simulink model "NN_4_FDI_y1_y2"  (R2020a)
settings: Solver=VariableStepAuto  StartTime=0.0  StopTime=30  RelTol=1e-3
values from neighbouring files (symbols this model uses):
  C = 6.3000e-04    (= 0.00063)    [maglev_init.m]
  g = 9.80    (= 9.8)    [maglev_init.m]
  K = 1.0e+03 * [-2.4567   -0.1235    0.0237]    [maglev_init.m]
  L1 = 0.6000    (= 0.6)    [maglev_init.m]
  m = 0.0300    (= 0.03)    [maglev_init.m]
  mpert = 0    [maglev_init.m]
  R = 45    [maglev_init.m]
  Ts = 0.005    [maglev_init.m]    (also in train_net.m)
  x1_0 = 0.1    [maglev_init.m]
  x1_d = 0.05    [maglev_init.m]
  x2_0 = 0    [maglev_init.m]
  x2_d = 0    [maglev_init.m]
  x3_0 = 0.2    [maglev_init.m]
libraries: neural x36

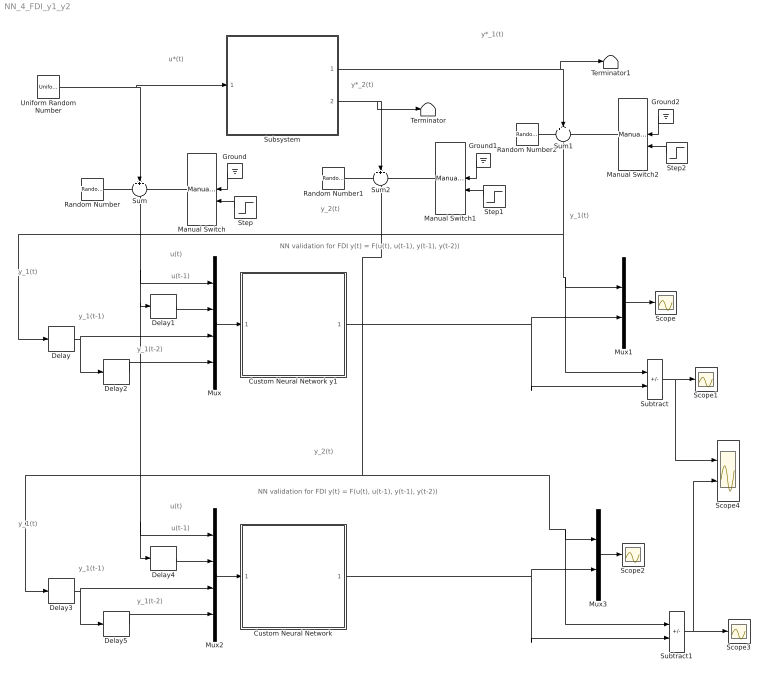
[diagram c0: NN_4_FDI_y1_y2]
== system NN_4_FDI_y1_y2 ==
  note: y_1(t)
  note: y_1(t-1)
  note: NN validation for FDI y(t) = F(u(t), u(t-1), y(t-1), y(t-2))
  note: y_2(t)
  note: y*_1(t)
  note: u(t)
  note: u*(t)
  note: y*_2(t)
  note: y_1(t)
  note: u(t-1)
  note: y_1(t-2)
  note: y_1(t)
  note: y_1(t-1)
  note: u(t-1)
  note: NN validation for FDI y(t) = F(u(t), u(t-1), y(t-1), y(t-2))
  note: u(t)
  note: y_1(t-2)
  note: y_2(t)
  Custom Neural Network : Subsystem
      mask help: Custom Neural Network
  Custom Neural Network y1 : Subsystem
      mask help: Custom Neural Network
  Delay{,1..5} (6 alike) : Delay  DelayLength=1  SampleTime=Ts
  Ground : Ground
  Ground1 : Ground
  Ground2 : Ground
  Manual Switch : ManualSwitch
  Manual Switch1 : ManualSwitch
  Manual Switch2 : ManualSwitch
  Mux : Mux
  Mux1 : Mux  Inputs=2
  Mux2 : Mux
  Mux3 : Mux  Inputs=2
  Random Number : RandomNumber  Variance=1e-9  Seed=1  SampleTime=Ts
  Random Number1 : RandomNumber  Variance=1e-6  Seed=3  SampleTime=Ts
  Random Number2 : RandomNumber  Variance=1e-9  Seed=2  SampleTime=Ts
  Scope{,1..3} (4 alike) : Scope
  Scope4 : Scope  NumInputPorts=2
  Step : Step  Time=15  SampleTime=0
  Step1 : Step  Time=15  After=5  SampleTime=0
  Step2 : Step  Time=15  SampleTime=0
  Subsystem : Subsystem
  Subtract : Sum  Inputs=+-
  Subtract1 : Sum  Inputs=+-
  Sum : Sum  Inputs=+++
  Sum1 : Sum  Inputs=+++
  Sum2 : Sum  Inputs=+++
  Terminator : Terminator
  Terminator1 : Terminator
  Uniform Random Number : UniformRandomNumber  Minimum=x1_d*0.9  Maximum=x1_d*1.1  Seed=1  SampleTime=0.5
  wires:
  Uniform Random Number/1 -> Subsystem/1(In1), Sum/2
  Subsystem/1(Out1) -> Terminator1/1, Sum1/2
  Subsystem/2(Out2) -> Terminator/1, Sum2/2
  Random Number/1 -> Sum/1
  Manual Switch/1 -> Sum/3
  Manual Switch2/1 -> Sum1/3
  Manual Switch1/1 -> Sum2/3
  Random Number1/1 -> Sum2/1
  Ground/1 -> Manual Switch/1
  Step/1 -> Manual Switch/2
  Ground1/1 -> Manual Switch1/1
  Step1/1 -> Manual Switch1/2
  Random Number2/1 -> Sum1/1
  Ground2/1 -> Manual Switch2/1
  Step2/1 -> Manual Switch2/2
  Sum1/1 -> Subtract/1, Mux1/1, Delay/1
  Delay1/1 -> Mux/2
  Delay/1 -> Delay2/1, Mux/3
  Delay2/1 -> Mux/4
  Mux/1 -> Custom Neural Network y1/1(Input)
  Custom Neural Network y1/1(Output) -> Subtract/2, Mux1/2
  Mux1/1 -> Scope/1
  Subtract/1 -> Scope4/1, Scope1/1
  Delay5/1 -> Mux2/4
  Mux3/1 -> Scope2/1
  Custom Neural Network/1(Output) -> Subtract1/2, Mux3/2
  Mux2/1 -> Custom Neural Network/1(Input)
  Delay3/1 -> Delay5/1, Mux2/3
  Sum/1 -> Delay4/1, Mux2/1, Delay1/1, Mux/1
  Delay4/1 -> Mux2/2
  Subtract1/1 -> Scope4/2, Scope3/1
  Sum2/1 -> Subtract1/1, Mux3/1, Delay3/1

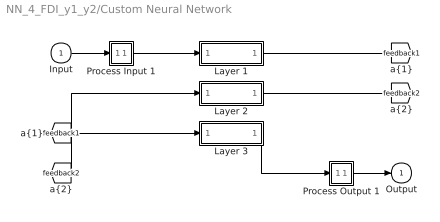
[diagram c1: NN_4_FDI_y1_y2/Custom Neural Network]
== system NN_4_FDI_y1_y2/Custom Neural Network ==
  Input : Inport  PortDimensions=4  SampleTime=0.005
  Layer 1 : Subsystem
  Layer 2 : Subsystem
  Layer 3 : Subsystem
  Process Input 1 : Subsystem
  Process Output 1 : Subsystem
  Output : Outport  InitialOutput=0
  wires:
  Input/1 -> Process Input 1/1(x)
  Process Output 1/1(y) -> Output/1
  Process Input 1/1(p) -> Layer 1/1("p{1}")
  Layer 1/1("a{1}") -> [feedback1]
  [feedback1] -> Layer 2/1("a{1} ")
  Layer 2/1("a{2}") -> [feedback2]
  [feedback2] -> Layer 3/1("a{2} ")
  Layer 3/1("a{3}") -> Process Output 1/1(a)

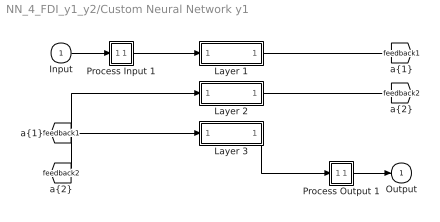
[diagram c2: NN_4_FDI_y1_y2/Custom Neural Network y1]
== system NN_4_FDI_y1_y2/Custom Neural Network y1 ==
  Input : Inport  PortDimensions=4  SampleTime=0.005
  Layer 1 : Subsystem
  Layer 2 : Subsystem
  Layer 3 : Subsystem
  Process Input 1 : Subsystem
  Process Output 1 : Subsystem
  Output : Outport  InitialOutput=0
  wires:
  Input/1 -> Process Input 1/1(x)
  Process Output 1/1(y) -> Output/1
  Process Input 1/1(p) -> Layer 1/1("p{1}")
  Layer 1/1("a{1}") -> [feedback1]
  [feedback1] -> Layer 2/1("a{1} ")
  Layer 2/1("a{2}") -> [feedback2]
  [feedback2] -> Layer 3/1("a{2} ")
  Layer 3/1("a{3}") -> Process Output 1/1(a)

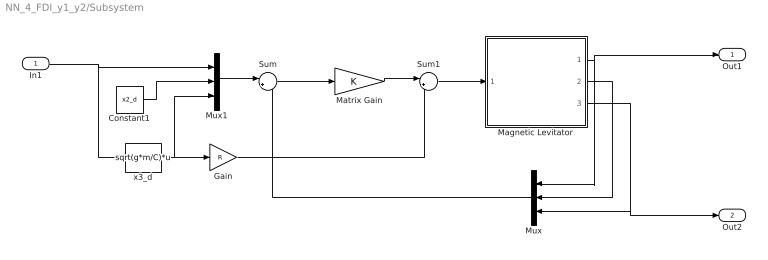
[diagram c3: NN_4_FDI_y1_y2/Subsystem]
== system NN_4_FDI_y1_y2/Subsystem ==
  In1 : Inport
  Constant1 : Constant  Value=x2_d
  Gain : Gain  Gain=R
  Magnetic Levitator : Subsystem  mask{m=m+mpert, R=R, L1=L1, C=C, g=g}
      mask prompts: m "ball's mass (m)"; R "Electromagnet's resistance (R)"; L1 "Electromagnet's inductance (L1)"; C "Magnetic force constant (C)"; g "Gravitational acceleration (g)"
  Matrix Gain : Gain  Gain=K  Multiplication=Matrix(K*u)  SaturateOnIntegerOverflow=on
  Mux : Mux  Inputs=3
  Mux1 : Mux  Inputs=3
  Sum : Sum  Inputs=|+-  InputSameDT=on  SaturateOnIntegerOverflow=on
  Sum1 : Sum  Inputs=|++  InputSameDT=on  SaturateOnIntegerOverflow=on
  x3_d : Fcn  Expr=sqrt(g*m/C)*u
  Out1 : Outport
  Out2 : Outport  Port=2
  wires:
  In1/1 -> x3_d/1, Mux1/1
  Magnetic Levitator/2(x2) -> Mux/2
  x3_d/1 -> Mux1/3, Gain/1
  Mux1/1 -> Sum/1
  Gain/1 -> Sum1/2
  Mux/1 -> Sum/2
  Constant1/1 -> Mux1/2
  Sum/1 -> Matrix Gain/1
  Sum1/1 -> Magnetic Levitator/1(u)
  Magnetic Levitator/1(x1) -> Out1/1, Mux/1
  Magnetic Levitator/3(x3) -> Out2/1, Mux/3
  Matrix Gain/1 -> Sum1/1

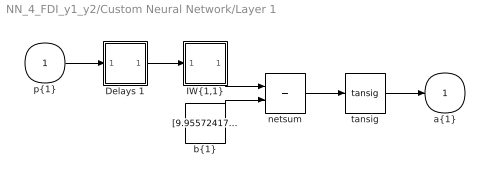
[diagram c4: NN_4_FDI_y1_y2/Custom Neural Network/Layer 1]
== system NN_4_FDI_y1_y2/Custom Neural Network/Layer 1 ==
  "p{1}" : Inport  PortDimensions=4  SampleTime=0.005
  Delays 1 : Subsystem
  "IW{1,1}" : Subsystem
  "b{1}" : Constant  Value=[9.9557241726304166462568900897167623043060302734375;10.8017518649547294984358813962899148464202880859375;3.779362190875286131586108240298926830291748046875;13.70534100885252115631374181248247623443603515625]
  netsum : Sum  Inputs=2  InputSameDT=on  SaturateOnIntegerOverflow=on
  tansig : neural/Transfer Functions/tansig
  "a{1}" : Outport  InitialOutput=[0;0;0;0]
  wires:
  "p{1}"/1 -> Delays 1/1("p{1}")
  Delays 1/1("pd{1,1}") -> "IW{1,1}"/1("pd{1,1}")
  "IW{1,1}"/1("iz{1,1}") -> netsum/1
  "b{1}"/1 -> netsum/2
  netsum/1 -> tansig/1
  tansig/1 -> "a{1}"/1

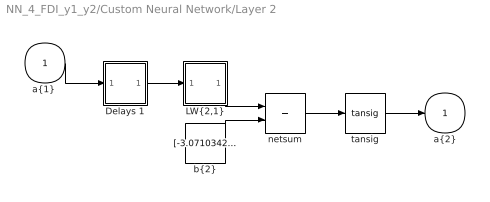
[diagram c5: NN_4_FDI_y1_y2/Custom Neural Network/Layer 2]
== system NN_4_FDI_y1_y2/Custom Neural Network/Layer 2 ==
  "a{1} " : Inport  PortDimensions=4  SampleTime=0.005
  Delays 1 : Subsystem
  "LW{2,1}" : Subsystem
  "b{2}" : Constant  Value=[-3.071034257137068568255244827014394104480743408203125;1.6519477133200834995108152725151740014553070068359375;2.0170506290868939203164700302295386791229248046875;-0.93388372923963192118179676981526426970958709716796875;0.3845725321207089653086086400435306131839752197265625;-0.39336279890520386981478395682643167674541473388671875;0.930508654862947093278080501477234065532684326171875;1.911370482300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
  netsum : Sum  Inputs=2  InputSameDT=on  SaturateOnIntegerOverflow=on
  tansig : neural/Transfer Functions/tansig
  "a{2}" : Outport  InitialOutput=[0;0;0;0;0;0;0;0;0;0]
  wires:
  "a{1} "/1 -> Delays 1/1("p{2}")
  Delays 1/1("pd{2,1}") -> "LW{2,1}"/1("ad{2,1}")
  "LW{2,1}"/1("lz{2,1}") -> netsum/1
  "b{2}"/1 -> netsum/2
  netsum/1 -> tansig/1
  tansig/1 -> "a{2}"/1

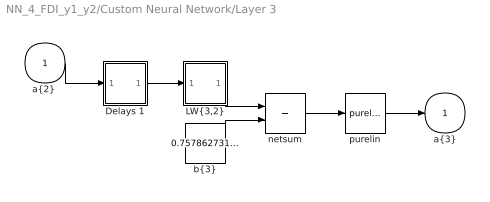
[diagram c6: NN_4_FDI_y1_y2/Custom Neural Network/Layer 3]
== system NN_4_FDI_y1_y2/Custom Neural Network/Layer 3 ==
  "a{2} " : Inport  PortDimensions=10  SampleTime=0.005
  Delays 1 : Subsystem
  "LW{3,2}" : Subsystem
  "b{3}" : Constant  Value=0.7578627315964741040232865998405031859874725341796875
  netsum : Sum  Inputs=2  InputSameDT=on  SaturateOnIntegerOverflow=on
  purelin : neural/Transfer Functions/purelin
  "a{3}" : Outport  InitialOutput=0
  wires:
  "a{2} "/1 -> Delays 1/1("p{3}")
  Delays 1/1("pd{3,2}") -> "LW{3,2}"/1("ad{3,2}")
  "LW{3,2}"/1("lz{3,2}") -> netsum/1
  "b{3}"/1 -> netsum/2
  netsum/1 -> purelin/1
  purelin/1 -> "a{3}"/1

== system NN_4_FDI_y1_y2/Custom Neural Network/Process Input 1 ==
  x : Inport  PortDimensions=4  SampleTime=0.005
  p : Outport  PortDimensions=4  SampleTime=0.005
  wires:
  x/1 -> p/1

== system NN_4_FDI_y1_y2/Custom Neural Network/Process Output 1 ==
  a : Inport  PortDimensions=1  SampleTime=0.005
  y : Outport  PortDimensions=1  SampleTime=0.005
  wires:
  a/1 -> y/1

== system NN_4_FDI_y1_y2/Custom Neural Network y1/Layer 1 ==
  "p{1}" : Inport  PortDimensions=4  SampleTime=0.005
  Delays 1 : Subsystem
  "IW{1,1}" : Subsystem
  "b{1}" : Constant  Value=[11.744601348517022643136442638933658599853515625;10.199640082309191058129727025516331195831298828125;-17.03232759988026856490250793285667896270751953125;13.5748992182948189366697988589294254779815673828125]
  netsum : Sum  Inputs=2  InputSameDT=on  SaturateOnIntegerOverflow=on
  tansig : neural/Transfer Functions/tansig
  "a{1}" : Outport  InitialOutput=[0;0;0;0]
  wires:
  "p{1}"/1 -> Delays 1/1("p{1}")
  Delays 1/1("pd{1,1}") -> "IW{1,1}"/1("pd{1,1}")
  "IW{1,1}"/1("iz{1,1}") -> netsum/1
  "b{1}"/1 -> netsum/2
  netsum/1 -> tansig/1
  tansig/1 -> "a{1}"/1

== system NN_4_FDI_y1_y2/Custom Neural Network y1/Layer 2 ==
  "a{1} " : Inport  PortDimensions=4  SampleTime=0.005
  Delays 1 : Subsystem
  "LW{2,1}" : Subsystem
  "b{2}" : Constant  Value=[2.514902413299356709330822923220694065093994140625;-1.905736181055616373924976869602687656879425048828125;-1.3244117236339700838243516045622527599334716796875;1.4169478908980768228076385639724321663379669189453125;-0.54494294986358460253228486180887557566165924072265625;0.1603376935224779253896798536516143940389156341552734375;-0.8398255160686165510242062737233936786651611328125;-1.30541599158430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
  netsum : Sum  Inputs=2  InputSameDT=on  SaturateOnIntegerOverflow=on
  tansig : neural/Transfer Functions/tansig
  "a{2}" : Outport  InitialOutput=[0;0;0;0;0;0;0;0;0;0]
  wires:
  "a{1} "/1 -> Delays 1/1("p{2}")
  Delays 1/1("pd{2,1}") -> "LW{2,1}"/1("ad{2,1}")
  "LW{2,1}"/1("lz{2,1}") -> netsum/1
  "b{2}"/1 -> netsum/2
  netsum/1 -> tansig/1
  tansig/1 -> "a{2}"/1

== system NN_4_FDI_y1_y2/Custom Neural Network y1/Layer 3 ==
  "a{2} " : Inport  PortDimensions=10  SampleTime=0.005
  Delays 1 : Subsystem
  "LW{3,2}" : Subsystem
  "b{3}" : Constant  Value=-0.57244236899128775331035967610660009086132049560546875
  netsum : Sum  Inputs=2  InputSameDT=on  SaturateOnIntegerOverflow=on
  purelin : neural/Transfer Functions/purelin
  "a{3}" : Outport  InitialOutput=0
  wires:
  "a{2} "/1 -> Delays 1/1("p{3}")
  Delays 1/1("pd{3,2}") -> "LW{3,2}"/1("ad{3,2}")
  "LW{3,2}"/1("lz{3,2}") -> netsum/1
  "b{3}"/1 -> netsum/2
  netsum/1 -> purelin/1
  purelin/1 -> "a{3}"/1

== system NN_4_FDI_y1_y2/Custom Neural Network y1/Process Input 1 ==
  x : Inport  PortDimensions=4  SampleTime=0.005
  p : Outport  PortDimensions=4  SampleTime=0.005
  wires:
  x/1 -> p/1

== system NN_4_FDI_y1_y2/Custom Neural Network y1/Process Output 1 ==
  a : Inport  PortDimensions=1  SampleTime=0.005
  y : Outport  PortDimensions=1  SampleTime=0.005
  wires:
  a/1 -> y/1

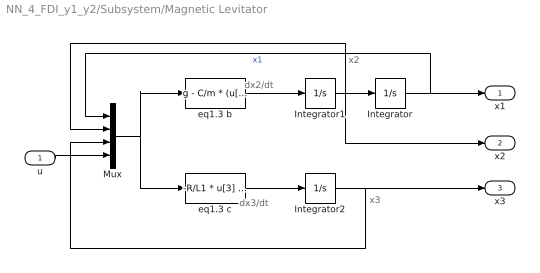
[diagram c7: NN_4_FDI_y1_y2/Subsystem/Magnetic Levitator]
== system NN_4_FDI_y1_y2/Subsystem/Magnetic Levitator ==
  note: x2
  note: x3
  note: dx2/dt
  note: dx3/dt
  u : Inport
  Integrator : Integrator  InitialCondition=x1_0
  Integrator1 : Integrator  InitialCondition=x2_0
  Integrator2 : Integrator  InitialCondition=x3_0
  Mux : Mux
  eq1.3 b : Fcn  Expr=g - C/m * (u[3] / u[1])^2
  eq1.3 c : Fcn  Expr=-R/L1 * u[3] + (2*C)/L1 * ( u[2] * u[3] / u[1]^2 ) + 1/L1 * u[4]
  x1 : Outport
  x2 : Outport  Port=2
  x3 : Outport  Port=3
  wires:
  eq1.3 b/1 -> Integrator1/1
  Integrator1/1 -> Integrator/1, Mux/2, x2/1
  eq1.3 c/1 -> Integrator2/1
  Mux/1 -> eq1.3 b/1, eq1.3 c/1
  Integrator/1 -> Mux/1, x1/1  "x1"
  Integrator2/1 -> Mux/3, x3/1
  u/1 -> Mux/4

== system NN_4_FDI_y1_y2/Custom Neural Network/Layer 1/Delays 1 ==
  "p{1}" : Inport  PortDimensions=4  SampleTime=0.005
  mux : Mux  Inputs=1
  "pd{1,1}" : Outport
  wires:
  "p{1}"/1 -> mux/1
  mux/1 -> "pd{1,1}"/1

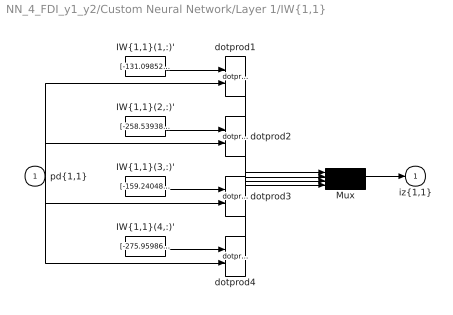
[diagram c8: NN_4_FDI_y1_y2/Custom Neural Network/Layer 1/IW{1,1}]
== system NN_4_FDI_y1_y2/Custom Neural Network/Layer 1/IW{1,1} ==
  "pd{1,1}" : Inport  PortDimensions=4  SampleTime=0.005
  "IW{1,1}(1,:)'" : Constant  Value=[-131.098527078192518047217163257300853729248046875;0.592044032651457552418605700950138270854949951171875;-2.12284817944854165006063340115360915660858154296875;0.5765404591733724881663647465757094323635101318359375]
  "IW{1,1}(2,:)'" : Constant  Value=[-258.539381892176834298879839479923248291015625;28.400775583851338268459585378877818584442138671875;-0.321276434762693074986827923567034304141998291015625;1.632418072873166092762176049291156232357025146484375]
  "IW{1,1}(3,:)'" : Constant  Value=[-159.24048115718187546008266508579254150390625;18.598481968734223102046598796732723712921142578125;3.02382446626069789630264494917355477809906005859375;-0.060921937687954348661367731665450264699757099151611328125]
  "IW{1,1}(4,:)'" : Constant  Value=[-275.95986358683086336895939894020557403564453125;-45.6117914706242544298220309428870677947998046875;-0.05999788421777972613480045538381091319024562835693359375;0.40478921567869929898364489417872391641139984130859375]
  Mux : Mux
  dotprod{1..4} (4 alike) : neural/Weight Functions/dotprod
  "iz{1,1}" : Outport
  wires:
  "IW{1,1}(1,:)'"/1 -> dotprod1/1
  "pd{1,1}"/1 -> dotprod1/2, dotprod2/2, dotprod3/2, dotprod4/2
  dotprod1/1 -> Mux/1
  "IW{1,1}(2,:)'"/1 -> dotprod2/1
  dotprod2/1 -> Mux/2
  "IW{1,1}(3,:)'"/1 -> dotprod3/1
  dotprod3/1 -> Mux/3
  "IW{1,1}(4,:)'"/1 -> dotprod4/1
  dotprod4/1 -> Mux/4
  Mux/1 -> "iz{1,1}"/1

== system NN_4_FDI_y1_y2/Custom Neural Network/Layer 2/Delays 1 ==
  "p{2}" : Inport  PortDimensions=4  SampleTime=0.005
  mux : Mux  Inputs=1
  "pd{2,1}" : Outport
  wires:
  "p{2}"/1 -> mux/1
  mux/1 -> "pd{2,1}"/1

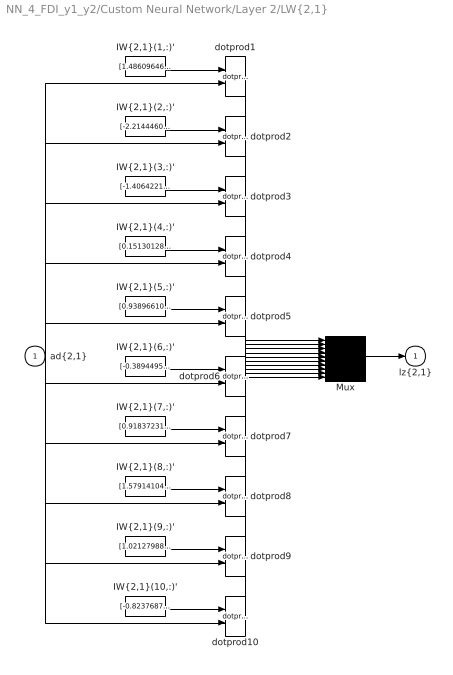
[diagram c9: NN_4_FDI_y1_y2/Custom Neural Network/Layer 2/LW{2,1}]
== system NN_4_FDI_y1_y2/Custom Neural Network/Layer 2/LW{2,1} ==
  "ad{2,1}" : Inport  PortDimensions=4  SampleTime=0.005
  "IW{2,1}(1,:)'" : Constant  Value=[1.4860964683035040589942354927188716828823089599609375;1.9682201340324312344165491595049388706684112548828125;0.093140637900932354842353788626496680080890655517578125;1.2926693086141745059336471967981196939945220947265625]
  "IW{2,1}(10,:)'" : Constant  Value=[-0.82376876991053393783914771120180375874042510986328125;-1.5110532368794695745606304626562632620334625244140625;1.7801107366741197868265089709893800318241119384765625;0.31935665794871403999621861657942645251750946044921875]
  "IW{2,1}(2,:)'" : Constant  Value=[-2.2144460785248103462663493701256811618804931640625;0.048235313777043258010035486904598656110465526580810546875;0.13631673272389466244902678226935677230358123779296875;-1.5046722770630740484421039582230150699615478515625]
  "IW{2,1}(3,:)'" : Constant  Value=[-1.4064221455699004170725174844847060739994049072265625;-0.6583003276452761287629300568369217216968536376953125;1.02805120094084312398763358942233026027679443359375;0.71569871268339013692383332454483024775981903076171875]
  "IW{2,1}(4,:)'" : Constant  Value=[0.1513012847034406471724565790282213129103183746337890625;-0.7206033750997227205203898847685195505619049072265625;1.0012141411901591681044010329060256481170654296875;-1.2696855067788812565510170315974391996860504150390625]
  "IW{2,1}(5,:)'" : Constant  Value=[0.938966102416004755326639497070573270320892333984375;1.50233182161680733912589857936836779117584228515625;0.7849663643621707098674278313410468399524688720703125;-2.388143748385829656655232611228711903095245361328125]
  "IW{2,1}(6,:)'" : Constant  Value=[-0.38944959823569436085932693458744324743747711181640625;0.39381299353723842049390668762498535215854644775390625;-2.06988324216109109698891188600100576877593994140625;1.299018407696672650075697674765251576900482177734375]
  "IW{2,1}(7,:)'" : Constant  Value=[0.9183723159364129973170065568410791456699371337890625;0.2152093714512781919001582764394697733223438262939453125;-2.041684926202248728799304444692097604274749755859375;-0.6481878502810973774472813602187670767307281494140625]
  "IW{2,1}(8,:)'" : Constant  Value=[1.579141043106157216158180744969286024570465087890625;1.1866613438782425138384724050411023199558258056640625;-1.5830475137551773823219036785303615033626556396484375;0.257682618814930763928572332588373683393001556396484375]
  "IW{2,1}(9,:)'" : Constant  Value=[1.0212798862014214051896487944759428501129150390625;-1.5473822547842412955532154228421859443187713623046875;1.191088307160548698249158405815251171588897705078125;0.75097654659082457850871605842257849872112274169921875]
  Mux : Mux  Inputs=10
  dotprod{1..10} (10 alike) : neural/Weight Functions/dotprod
  "lz{2,1}" : Outport
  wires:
  "IW{2,1}(1,:)'"/1 -> dotprod1/1
  "ad{2,1}"/1 -> dotprod1/2, dotprod2/2, dotprod3/2, dotprod4/2, dotprod5/2, dotprod6/2, dotprod7/2, dotprod8/2, dotprod9/2, dotprod10/2
  dotprod1/1 -> Mux/1
  "IW{2,1}(2,:)'"/1 -> dotprod2/1
  dotprod2/1 -> Mux/2
  "IW{2,1}(3,:)'"/1 -> dotprod3/1
  dotprod3/1 -> Mux/3
  "IW{2,1}(4,:)'"/1 -> dotprod4/1
  dotprod4/1 -> Mux/4
  "IW{2,1}(5,:)'"/1 -> dotprod5/1
  dotprod5/1 -> Mux/5
  "IW{2,1}(6,:)'"/1 -> dotprod6/1
  dotprod6/1 -> Mux/6
  "IW{2,1}(7,:)'"/1 -> dotprod7/1
  dotprod7/1 -> Mux/7
  "IW{2,1}(8,:)'"/1 -> dotprod8/1
  dotprod8/1 -> Mux/8
  "IW{2,1}(9,:)'"/1 -> dotprod9/1
  dotprod9/1 -> Mux/9
  "IW{2,1}(10,:)'"/1 -> dotprod10/1
  dotprod10/1 -> Mux/10
  Mux/1 -> "lz{2,1}"/1

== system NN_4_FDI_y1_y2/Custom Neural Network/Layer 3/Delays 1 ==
  "p{3}" : Inport  PortDimensions=10  SampleTime=0.005
  mux : Mux  Inputs=1
  "pd{3,2}" : Outport
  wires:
  "p{3}"/1 -> mux/1
  mux/1 -> "pd{3,2}"/1

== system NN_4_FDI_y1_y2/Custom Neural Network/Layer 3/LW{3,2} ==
  "ad{3,2}" : Inport  PortDimensions=10  SampleTime=0.005
  "IW{3,2}(1,:)'" : Constant  Value=[-0.83644295544000779596416350614163093268871307373046875;-0.6774391217628179528986720470129512250423431396484375;0.242857323721097750901520839761360548436641693115234375;0.1915070686106929709335844336237641982734203338623046875;0.79549203850041771968193415887071751058101654052734375;-0.3606304077624855608519283123314380645751953125;-0.51533634861189525633307084717671386897563934326171875;-0.54711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
  Mux : Mux  Inputs=1
  dotprod1 : neural/Weight Functions/dotprod
  "lz{3,2}" : Outport
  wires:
  "IW{3,2}(1,:)'"/1 -> dotprod1/1
  "ad{3,2}"/1 -> dotprod1/2
  dotprod1/1 -> Mux/1
  Mux/1 -> "lz{3,2}"/1

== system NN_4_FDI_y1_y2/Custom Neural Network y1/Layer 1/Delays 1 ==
  "p{1}" : Inport  PortDimensions=4  SampleTime=0.005
  mux : Mux  Inputs=1
  "pd{1,1}" : Outport
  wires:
  "p{1}"/1 -> mux/1
  mux/1 -> "pd{1,1}"/1

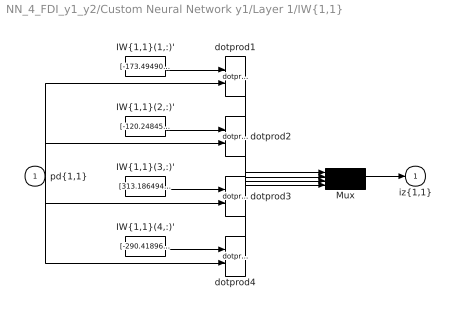
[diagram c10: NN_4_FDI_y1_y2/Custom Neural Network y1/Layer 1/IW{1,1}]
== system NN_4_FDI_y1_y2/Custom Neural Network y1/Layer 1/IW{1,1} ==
  "pd{1,1}" : Inport  PortDimensions=4  SampleTime=0.005
  "IW{1,1}(1,:)'" : Constant  Value=[-173.494909352381085909655666910111904144287109375;-54.70106297212252144390731700696051120758056640625;9.6305050168924939413273023092187941074371337890625;16.0477816031816900022022309713065624237060546875]
  "IW{1,1}(2,:)'" : Constant  Value=[-120.24845524473670366205624304711818695068359375;-49.60338222643863304028855054639279842376708984375;-3.941136589596483386088721090345643460750579833984375;-25.36364173271520172647797153331339359283447265625]
  "IW{1,1}(3,:)'" : Constant  Value=[313.186494358965092033031396567821502685546875;26.592748444340482905090539134107530117034912109375;4.3443123180997940124825618113391101360321044921875;18.35151034836506056535654352046549320220947265625]
  "IW{1,1}(4,:)'" : Constant  Value=[-290.41896729500666651802021078765392303466796875;25.411409156004584275478919153101742267608642578125;-12.35088197055370784482875023968517780303955078125;-18.834304615077950728618816356174647808074951171875]
  Mux : Mux
  dotprod{1..4} (4 alike) : neural/Weight Functions/dotprod
  "iz{1,1}" : Outport
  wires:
  "IW{1,1}(1,:)'"/1 -> dotprod1/1
  "pd{1,1}"/1 -> dotprod1/2, dotprod2/2, dotprod3/2, dotprod4/2
  dotprod1/1 -> Mux/1
  "IW{1,1}(2,:)'"/1 -> dotprod2/1
  dotprod2/1 -> Mux/2
  "IW{1,1}(3,:)'"/1 -> dotprod3/1
  dotprod3/1 -> Mux/3
  "IW{1,1}(4,:)'"/1 -> dotprod4/1
  dotprod4/1 -> Mux/4
  Mux/1 -> "iz{1,1}"/1

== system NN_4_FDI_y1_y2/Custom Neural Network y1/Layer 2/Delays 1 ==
  "p{2}" : Inport  PortDimensions=4  SampleTime=0.005
  mux : Mux  Inputs=1
  "pd{2,1}" : Outport
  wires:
  "p{2}"/1 -> mux/1
  mux/1 -> "pd{2,1}"/1

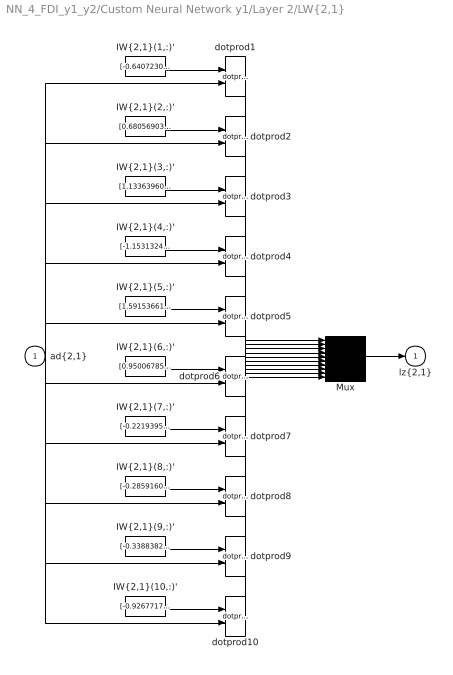
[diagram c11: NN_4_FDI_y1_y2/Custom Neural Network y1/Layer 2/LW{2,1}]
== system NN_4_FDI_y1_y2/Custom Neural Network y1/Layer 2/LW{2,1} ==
  "ad{2,1}" : Inport  PortDimensions=4  SampleTime=0.005
  "IW{2,1}(1,:)'" : Constant  Value=[-0.64072307351987489720812618543277494609355926513671875;-0.03196781043370389152613597616436891257762908935546875;1.8816722496400359876389529745210893452167510986328125;-1.4798868410796630623593728159903548657894134521484375]
  "IW{2,1}(10,:)'" : Constant  Value=[-0.9267717038632434789491298943175934255123138427734375;1.1709023012586519119082595352665521204471588134765625;-1.0258546733481790358410989938420243561267852783203125;1.5846434428193585386424047101172618567943572998046875]
  "IW{2,1}(2,:)'" : Constant  Value=[0.68056903784166744575401253314339555799961090087890625;0.05348767084577173147597051183765870518982410430908203125;0.56798527366561923912513520917855203151702880859375;-2.24531995696636155201986184692941606044769287109375]
  "IW{2,1}(3,:)'" : Constant  Value=[1.13363960568859400979135898523963987827301025390625;1.6471231374235213440471170542878098785877227783203125;0.3548356881963778963751110495650209486484527587890625;-1.0941388067152180152419305159128271043300628662109375]
  "IW{2,1}(4,:)'" : Constant  Value=[-1.15313245852581314210283380816690623760223388671875;1.3651076719469241727011876719188876450061798095703125;0.44703169752749527532387219252996146678924560546875;-0.60684098679539577592123578142491169273853302001953125]
  "IW{2,1}(5,:)'" : Constant  Value=[1.5915366156900818683794796015718020498752593994140625;0.54246774690524046658168799694976769387722015380859375;-1.54283519483922848536394667462445795536041259765625;-0.64038214037054019822647887849598191678524017333984375]
  "IW{2,1}(6,:)'" : Constant  Value=[0.95006785779222069354688073872239328920841217041015625;0.0305932799232624640095590251576140872202813625335693359375;-0.67661907381603436650863159229629673063755035400390625;1.929246258981040629265635288902558386325836181640625]
  "IW{2,1}(7,:)'" : Constant  Value=[-0.2219395023323143811833091376684023998677730560302734375;2.439162337071193231707866289070807397365570068359375;-0.2185872444755941612637428761445335112512111663818359375;-0.5234325157383012960821133674471639096736907958984375]
  "IW{2,1}(8,:)'" : Constant  Value=[-0.285916081769056529271466615682584233582019805908203125;0.1493805857291446714807392481816350482404232025146484375;-1.1450641138770356608489464633748866617679595947265625;-2.235874570960201257463495494448579847812652587890625]
  "IW{2,1}(9,:)'" : Constant  Value=[-0.338838292628626358560239850703510455787181854248046875;-0.21320513151665909656884423384326510131359100341796875;1.6112631364277998358147669932805001735687255859375;1.8120314381120063984553780755959451198577880859375]
  Mux : Mux  Inputs=10
  dotprod{1..10} (10 alike) : neural/Weight Functions/dotprod
  "lz{2,1}" : Outport
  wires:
  "IW{2,1}(1,:)'"/1 -> dotprod1/1
  "ad{2,1}"/1 -> dotprod1/2, dotprod2/2, dotprod3/2, dotprod4/2, dotprod5/2, dotprod6/2, dotprod7/2, dotprod8/2, dotprod9/2, dotprod10/2
  dotprod1/1 -> Mux/1
  "IW{2,1}(2,:)'"/1 -> dotprod2/1
  dotprod2/1 -> Mux/2
  "IW{2,1}(3,:)'"/1 -> dotprod3/1
  dotprod3/1 -> Mux/3
  "IW{2,1}(4,:)'"/1 -> dotprod4/1
  dotprod4/1 -> Mux/4
  "IW{2,1}(5,:)'"/1 -> dotprod5/1
  dotprod5/1 -> Mux/5
  "IW{2,1}(6,:)'"/1 -> dotprod6/1
  dotprod6/1 -> Mux/6
  "IW{2,1}(7,:)'"/1 -> dotprod7/1
  dotprod7/1 -> Mux/7
  "IW{2,1}(8,:)'"/1 -> dotprod8/1
  dotprod8/1 -> Mux/8
  "IW{2,1}(9,:)'"/1 -> dotprod9/1
  dotprod9/1 -> Mux/9
  "IW{2,1}(10,:)'"/1 -> dotprod10/1
  dotprod10/1 -> Mux/10
  Mux/1 -> "lz{2,1}"/1

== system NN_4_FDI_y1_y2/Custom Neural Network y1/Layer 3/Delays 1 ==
  "p{3}" : Inport  PortDimensions=10  SampleTime=0.005
  mux : Mux  Inputs=1
  "pd{3,2}" : Outport
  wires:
  "p{3}"/1 -> mux/1
  mux/1 -> "pd{3,2}"/1

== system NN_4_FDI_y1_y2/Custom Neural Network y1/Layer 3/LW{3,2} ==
  "ad{3,2}" : Inport  PortDimensions=10  SampleTime=0.005
  "IW{3,2}(1,:)'" : Constant  Value=[-0.0203064325877122288377396586156464763917028903961181640625;-0.10624673317698744845483105336825246922671794891357421875;-0.00520654423384775584537909054461124469526112079620361328125;-0.0759995107900031940939555852310149930417537689208984375;0.0301253913024823703759036419569383724592626094818115234375;-0.10909826716373173527419027095675119198858737945556640625;-0.0158214061333444046264506965826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
  Mux : Mux  Inputs=1
  dotprod1 : neural/Weight Functions/dotprod
  "lz{3,2}" : Outport
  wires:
  "IW{3,2}(1,:)'"/1 -> dotprod1/1
  "ad{3,2}"/1 -> dotprod1/2
  dotprod1/1 -> Mux/1
  Mux/1 -> "lz{3,2}"/1
